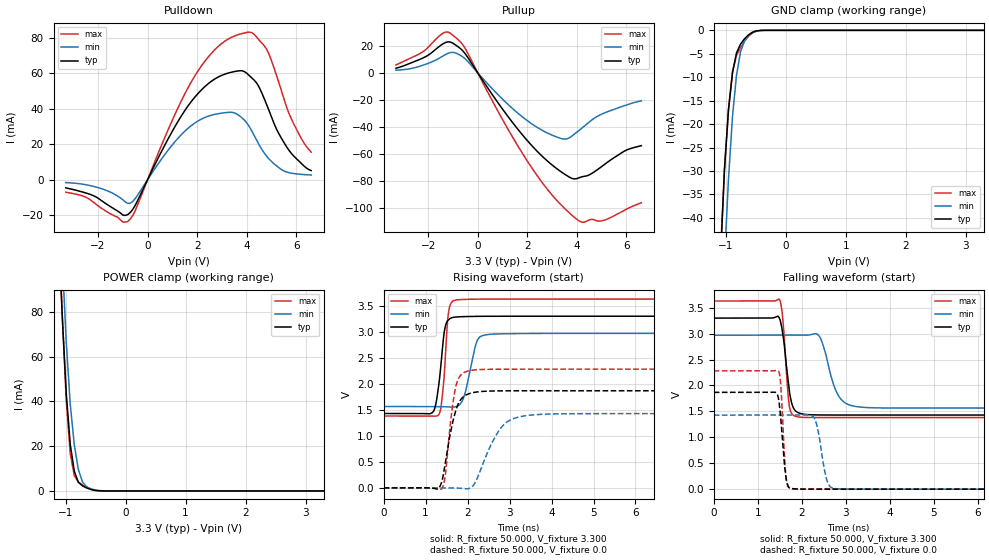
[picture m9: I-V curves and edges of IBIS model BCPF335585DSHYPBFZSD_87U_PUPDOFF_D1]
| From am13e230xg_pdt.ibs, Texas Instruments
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|   Model BCPF335585DSHYPBFZSD_87U_PUPDOFF_D1
[Model] BCPF335585DSHYPBFZSD_87U_PUPDOFF_D1
Model_type I/O
Polarity   Non-Inverting
Enable   Active-Low
Vinl =  0.990V
Vinh =  2.310V
Vmeas =  1.650V
C_comp   0.826pF   0.766pF   0.903pF
[Model Spec]
Vinh   2.310V   2.079V   2.541V
Vinl   0.990V   0.891V   1.089V
Vmeas   1.650V   1.485V   1.815V
[Temperature Range]   25.000   0.155k   -40.000
[Voltage Range]   3.300V   2.970V   3.630V
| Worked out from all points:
|   slope of the pulldown table from 0 to 0.495 V, typ, clamps not added: 35.2 ohm
|   slope of the pullup table from 0 to 0.495 V, typ, clamps not added: 36.4 ohm
|   GND clamp passes 1 mA (typ) near -0.62 V on its own axis
|   POWER clamp passes 1 mA (typ) near -0.61 V on its own axis
|   rising waveform, R_fixture 50.000, V_fixture 3.300: 20-80 % time 150ps typ, 225ps min, 114ps max; typ from 1.43 V to 3.3 V
|   rising waveform, R_fixture 50.000, V_fixture 0.0: 20-80 % time 274ps typ, 503ps min, 192ps max; typ from 0 V to 1.87 V
|   falling waveform, R_fixture 50.000, V_fixture 3.300: 20-80 % time 154ps typ, 290ps min, 108ps max; typ from 3.3 V to 1.43 V
|   falling waveform, R_fixture 50.000, V_fixture 0.0: 20-80 % time 109ps typ, 170ps min, 83.7ps max; typ from 1.87 V to 0 V
[Pulldown]
|Voltage   I(typ)   I(min)   I(max)
-3.3V     -4.614mA   -1.634mA   -7.048mA
-1.8V     -12.39mA   -5.352mA   -16.63mA
-800mV    -19.66mA   -13.38mA   -23.53mA
-500mV    -14.47mA   -10.67mA   -17.48mA
900mV     24.84mA    17.92mA    30.43mA
1.9V      46.39mA    31.84mA    58.31mA
3.3V      60.22mA    37.94mA    79.55mA
4V        59.94mA    31.97mA    82.91mA
4.4V      54.41mA    22.2mA     80.28mA
4.8V      42.35mA    13.25mA    73.5mA
5.7V      16.58mA    3.955mA    37.36mA
6.6V      5.118mA    2.644mA    15.48mA
[Pullup]
|Voltage   I(typ)   I(min)   I(max)
-3.3V     3.377mA    1.874mA    5.808mA
-2.2V     11.01mA    5.664mA    15.66mA
-1.4V     21.36mA    12.47mA    29.22mA
-1.1V     22.68mA    14.94mA    29.14mA
-500mV    13.95mA    10.2mA     17.81mA
1V        -26.77mA   -19.43mA   -34.48mA
2.2V      -54.08mA   -37.91mA   -70.65mA
3.4V      -73.49mA   -48.65mA   -98.18mA
3.8V      -77.91mA   -46.61mA   -105.1mA
4.2V      -76.72mA   -40.82mA   -110.2mA
5V        -69.15mA   -30.48mA   -109.2mA
6.6V      -53.76mA   -20.65mA   -95.84mA
[GND_clamp]
|Voltage   I(typ)   I(min)   I(max)
-3.3V     -1.05A     -924.6mA   -1.319A
-1.089V   -48.91mA   -69.18mA   -47.99mA
-1.022V   -29.79mA   -49.12mA   -29.48mA
-955mV    -16.94mA   -31.76mA   -17.01mA
-888mV    -9.058mA   -18.35mA   -8.783mA
-821mV    -4.809mA   -9.52mA    -5.378mA
-754mV    -2.93mA    -4.589mA   -3.691mA
-687mV    -1.795mA   -2.237mA   -2.338mA
-620mV    -951.1uA   -1.117mA   -1.252mA
-553mV    -382.8uA   -509uA     -513.2uA
-352mV    -2.13uA    -12.42uA   -2.39uA
3.3V      0A         0A         0A
[POWER_clamp]
|Voltage   I(typ)   I(min)   I(max)
-3.3V     1.851A     2.08A      1.997A
-1.122V   119.7mA    148.8mA    125.5mA
-1.055V   78.16mA    104.2mA    79.19mA
-988mV    43.66mA    66.59mA    40.55mA
-921mV    20.7mA     38.68mA    16.69mA
-854mV    8.846mA    20.65mA    6.818mA
-787mV    3.933mA    9.757mA    4.019mA
-720mV    2.311mA    4.145mA    2.698mA
-653mV    1.397mA    1.942mA    1.618mA
-519mV    286.9uA    510.4uA    258.6uA
-318mV    2.223uA    16.05uA    1.035uA
3.3V      0A         0A         0A
[Ramp]
| variable   typ   min   max
dV/dt_r   1.120/0.274n   0.857/0.503n   1.369/0.192n
dV/dt_f   1.122/0.154n   0.843/0.289n   1.349/0.108n
R_load = 50.000
[Rising Waveform]
R_fixture= 50.000
V_fixture= 3.300
V_fixture_min= 2.970
V_fixture_max= 3.630
|time   V(typ)   V(min)   V(max)
0s        1.43V      1.564V     1.381V
1.141ns   1.437V     1.564V     1.382V
1.321ns   2.03V      1.563V     1.417V
1.417ns   2.817V     1.562V     1.915V
1.545ns   3.232V     1.557V     3.373V
1.744ns   3.286V     1.567V     3.614V
1.923ns   3.293V     1.774V     3.623V
2.23ns    3.298V     2.833V     3.628V
2.544ns   3.299V     2.953V     3.63V
25ns      3.3V       2.97V      3.63V
[Rising Waveform]
R_fixture= 50.000
V_fixture= 0.0
V_fixture_min= 0.0
V_fixture_max= 0.0
|time   V(typ)   V(min)   V(max)
0s        791.6nV    826.4nV    734.7nV
1.281ns   -24.12mV   457.6uV    -6.984mV
1.389ns   129.9mV    614.8uV    -17.13mV
1.462ns   442mV      770.9uV    201.1mV
1.61ns    1.133V     347.7uV    1.385V
1.727ns   1.507V     -2.27mV    1.97V
2.14ns    1.834V     51mV       2.266V
2.826ns   1.865V     1.185V     2.282V
3.626ns   1.867V     1.407V     2.282V
25ns      1.867V     1.428V     2.282V
[Falling Waveform]
R_fixture= 50.000
V_fixture= 3.300
V_fixture_min= 2.970
V_fixture_max= 3.630
|time   V(typ)   V(min)   V(max)
0s        3.3V       2.97V      3.63V
1.489ns   3.303V     2.97V      3.663V
1.565ns   3.011V     2.97V      3.308V
1.719ns   1.878V     2.97V      1.588V
1.806ns   1.573V     2.97V      1.426V
1.947ns   1.465V     2.97V      1.39V
2.381ns   1.431V     2.967V     1.381V
2.838ns   1.43V      1.796V     1.381V
3.396ns   1.43V      1.579V     1.381V
25ns      1.43V      1.564V     1.381V
[Falling Waveform]
R_fixture= 50.000
V_fixture= 0.0
V_fixture_min= 0.0
V_fixture_max= 0.0
|time   V(typ)   V(min)   V(max)
0s        1.867V     1.428V     2.282V
1.472ns   1.74V      1.428V     2.277V
1.526ns   1.328V     1.428V     1.951V
1.611ns   423.7mV    1.428V     549.4mV
1.646ns   189mV      1.428V     194.7mV
1.8ns     9.081mV    1.428V     7.001mV
2.288ns   198.3uV    1.364V     59.26uV
2.572ns   38.52uV    164.6mV    14.25uV
2.779ns   17.08uV    8.982mV    9.104uV
25ns      252.1nV    585.2nV    270.7nV
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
